|Texas Instruments Incorporated
|High-Speed Differential Line Tranceivers
|IBIS Model for SN65LVDM1676 and SN65LVDM1677
|Valid for datarates upto 650Mbps for transmitters and 200Mbps for Receivers
|Marketing part#   Voltage Range   Package-type   #pins/pkg-type
|SN65LVDM1676DGG   3.0V - 3.6V   TSSOP   64-pin(DGG) TSSOP
|SN65LVDM1676DGGG4   3.0V - 3.6V   TSSOP   64-pin(DGG) TSSOP
|SN65LVDM1676DGGR   3.0V - 3.6V   TSSOP   64-pin(DGG) TSSOP
|SN65LVDM1676DGGRG4   3.0V - 3.6V   TSSOP   64-pin(DGG) TSSOP
|SN65LVDM1677DGG   3.0V - 3.6V   TSSOP   64-pin(DGG) TSSOP
|SN65LVDM1677DGGG4   3.0V - 3.6V   TSSOP   64-pin(DGG) TSSOP
|SN65LVDM1677DGGR   3.0V - 3.6V   TSSOP   64-pin(DGG) TSSOP
|SN65LVDM1677DGGRG4   3.0V - 3.6V   TSSOP   64-pin(DGG) TSSOP
[IBIS Ver]   4.0
[File name]   sn65lvdm1676_77.ibs
[File Rev]   1.1
[Date]   01/30/2009
[Source]   Texas Instruments Incorporated.
   Analog-eLab, HPA
   12500 TI Blvd
   Dallas, TX -75243
   For Support e-mail: elab_ibis@list.ti.com
[Notes]   Revision History
   Rev 2.0: 05/09/2006
   - Initial Revision not matched to silicon
   - Revision to correct DC end points
   Rev 1.1: 01/30/2009
   - Revision is numbered down to 1.1, to comply with IBIS
   standard way of 1.x for models that are not matched to silicon
   - Models included for all the three corners
   - Models valid for SN65LVD1676 and SN65LVDM1677
   - Updated timing specficatio values for DIFF_BI and TTL_BI models
[Disclaimer] This model is designed as an aid for customers of Texas Instruments.
 TI and its licensors and suppliers make no warranties, either expressed
 or implied, with respect to this  model, including the warranties of
 merchantability or fitness for a particular purpose.
 The model is provided solely on an "as is" basis. The entire risk as to
 its quality and performance is with the customer.
[Copyright] (C)Copyright 2009 Texas Instruments Incorporated. All rights reserved.
|   SN65LVDM1676DGG, with no termination between xxY and xxZ
[Component]   SN65LVDM1676DGG
[Manufacturer]  Texas Instruments Incorporated
[Package]   |64-pin TSSOP
|   typ   min   max
R_pkg   0.3357   0.2722   0.3992
L_pkg   3.6063nH   2.3128nH   4.8998nH
C_pkg   0.7109pF   0.3688pF   1.0529pF
[Pin] signal_name  model_name   R_pin   L_pin   C_pin
 1   GND   GND   0.22128  4.47324nH  1.01397pF
 2   VCC   POWER   0.38744  4.54017nH  1.04184pF
 3   VCC   POWER   0.38686  4.26675nH  0.93417pF
 4   GND   GND   0.38300  3.98994nH  0.83251pF
 5   ATX/RX   ENABLE   0.38411  3.73937nH  0.73901pF
 6   A1A   TTL_BI   0.38160  3.47970nH  0.64411pF
 7   A2A   TTL_BI   0.37105  3.18719nH  0.49035pF
 8   A3A   TTL_BI   0.33642  2.84375nH  0.45074pF
 9   A4A   TTL_BI   0.30420  2.59359nH  0.45718pF
10   BTX/RX   ENABLE   0.30070  2.55030nH  0.46530pF
11   B1A   TTL_BI   0.27412  2.38775nH  0.44423pF
12   B2A   TTL_BI   0.28316  2.43458nH  0.43792pF
13   B3A   TTL_BI   0.28981  2.46842nH  0.44090pF
14   B4A   TTL_BI   0.28000  2.36957nH  0.41787pF
15   GND   GND   0.27427  2.26725nH  0.40273pF
16   VCC   POWER   0.27344  2.24702nH  0.36695pF
17   VCC   POWER   0.27230  2.24050nH  0.36679pF
18   GND   GND   0.27273  2.25890nH  0.40223pF
19   C1A   TTL_BI   0.27551  2.34562nH  0.41523pF
20   C2A   TTL_BI   0.27964  2.41073nH  0.43742pF
21   C3A   TTL_BI   0.27218  2.37082nH  0.43941pF
22   C4A   TTL_BI   0.28848  2.47629nH  0.45088pF
23   CTX/RX   ENABLE   0.30740  2.59389nH  0.46881pF
24   D1A   TTL_BI   0.34088  2.82097nH  0.46717pF
25   D2A   TTL_BI   0.34051  2.87482nH  0.44992pF
26   D3A   TTL_BI   0.37271  3.20165nH  0.49086pF
27   D4A   TTL_BI   0.37589  3.44878nH  0.64437pF
28   DTX/RX   ENABLE   0.37739  3.70266nH  0.74218pF
29   GND   GND   0.37850  3.96797nH  0.83809pF
30   VCC   POWER   0.38033  4.23320nH  0.94059pF
31   VCC   POWER   0.38354  4.52417nH  1.05059pF
32   GND   GND   0.21987  4.45173nH  1.01894pF
33   D4Z   DIFF_BI   0.38723  4.87938nH  0.97220pF
34   D4Y   DIFF_BI   0.38394  4.52468nH  1.04044pF
35   D3Z   DIFF_BI   0.38248  4.24575nH  0.93538pF
36   D3Y   DIFF_BI   0.38370  3.99984nH  0.83632pF
37   D2Z   DIFF_BI   0.38672  3.76077nH  0.74367pF
38   D2Y   DIFF_BI   0.39239  3.55100nH  0.65111pF
39   D1Z   DIFF_BI   0.38504  3.27768nH  0.49727pF
40   D1Y   DIFF_BI   0.31818  2.73755nH  0.44436pF
41   C4Z   DIFF_BI   0.32127  2.70100nH  0.45913pF
42   C4Y   DIFF_BI   0.31115  2.61731nH  0.46671pF
43   C3Z   DIFF_BI   0.30136  2.55465nH  0.45112pF
44   C3Y   DIFF_BI   0.29406  2.50298nH  0.44285pF
45   C2Z   DIFF_BI   0.29101  2.47812nH  0.44091pF
46   C2Y   DIFF_BI   0.28926  2.42717nH  0.41837pF
47   C1Z   DIFF_BI   0.28865  2.35505nH  0.40495pF
48   C1Y   DIFF_BI   0.28916  2.34232nH  0.36962pF
49   B4Z   DIFF_BI   0.28633  2.32500nH  0.36878pF
50   B4Y   DIFF_BI   0.28177  2.31280nH  0.40298pF
51   B3Z   DIFF_BI   0.27796  2.35941nH  0.41458pF
52   B3Y   DIFF_BI   0.27453  2.37863nH  0.43615pF
53   B2Z   DIFF_BI   0.27226  2.36951nH  0.43902pF
54   B2Y   DIFF_BI   0.27640  2.40099nH  0.44636pF
55   B1Z   DIFF_BI   0.29100  2.49139nH  0.46130pF
56   B1Y   DIFF_BI   0.29972  2.56747nH  0.45350pF
57   A4Z   DIFF_BI   0.32271  2.76232nH  0.44507pF
58   A4Y   DIFF_BI   0.39212  3.31525nH  0.49929pF
59   A3Z   DIFF_BI   0.39916  3.58578nH  0.65712pF
60   A3Y   DIFF_BI   0.39255  3.78985nH  0.75190pF
61   A2Z   DIFF_BI   0.38864  4.02433nH  0.84518pF
62   A2Y   DIFF_BI   0.38679  4.26678nH  0.94612pF
63   A1Z   DIFF_BI   0.38755  4.54277nH  1.05293pF
64   A1Y   DIFF_BI   0.39081  4.89981nH  0.97900pF
[Diff_pin]   inv_pin   vdiff   tdelay_typ   tdelay_min   tdelay_max
| The 'xxY' pin is diff_pin and the 'xxZ' pin is the inv_pin
34   33   100mV   0   0   0
36   35   100mV   0   0   0
38   37   100mV   0   0   0
40   39   100mV   0   0   0
42   41   100mV   0   0   0
44   43   100mV   0   0   0
46   45   100mV   0   0   0
48   47   100mV   0   0   0
50   49   100mV   0   0   0
52   51   100mV   0   0   0
54   53   100mV   0   0   0
56   55   100mV   0   0   0
58   57   100mV   0   0   0
60   59   100mV   0   0   0
62   61   100mV   0   0   0
64   63   100mV   0   0   0
|   SN65LVDM1677DGG, with 100 Ohm termination between xxY and xxZ
[Component]   SN65LVDM1677DGG
[Manufacturer]  Texas Instruments Incorporated
[Package]   |64-pin TSSOP
|   typ   min   max
R_pkg   0.3357   0.2722   0.3992
L_pkg   3.6063nH   2.3128nH   4.8998nH
C_pkg   0.7109pF   0.3688pF   1.0529pF
[Pin] signal_name  model_name   R_pin   L_pin   C_pin
 1   GND   GND   0.22128  4.47324nH  1.01397pF
 2   VCC   POWER   0.38744  4.54017nH  1.04184pF
 3   VCC   POWER   0.38686  4.26675nH  0.93417pF
 4   GND   GND   0.38300  3.98994nH  0.83251pF
 5   ATX/RX   ENABLE   0.38411  3.73937nH  0.73901pF
 6   A1A   TTL_BI   0.38160  3.47970nH  0.64411pF
 7   A2A   TTL_BI   0.37105  3.18719nH  0.49035pF
 8   A3A   TTL_BI   0.33642  2.84375nH  0.45074pF
 9   A4A   TTL_BI   0.30420  2.59359nH  0.45718pF
10   BTX/RX   ENABLE   0.30070  2.55030nH  0.46530pF
11   B1A   TTL_BI   0.27412  2.38775nH  0.44423pF
12   B2A   TTL_BI   0.28316  2.43458nH  0.43792pF
13   B3A   TTL_BI   0.28981  2.46842nH  0.44090pF
14   B4A   TTL_BI   0.28000  2.36957nH  0.41787pF
15   GND   GND   0.27427  2.26725nH  0.40273pF
16   VCC   POWER   0.27344  2.24702nH  0.36695pF
17   VCC   POWER   0.27230  2.24050nH  0.36679pF
18   GND   GND   0.27273  2.25890nH  0.40223pF
19   C1A   TTL_BI   0.27551  2.34562nH  0.41523pF
20   C2A   TTL_BI   0.27964  2.41073nH  0.43742pF
21   C3A   TTL_BI   0.27218  2.37082nH  0.43941pF
22   C4A   TTL_BI   0.28848  2.47629nH  0.45088pF
23   CTX/RX   ENABLE   0.30740  2.59389nH  0.46881pF
24   D1A   TTL_BI   0.34088  2.82097nH  0.46717pF
25   D2A   TTL_BI   0.34051  2.87482nH  0.44992pF
26   D3A   TTL_BI   0.37271  3.20165nH  0.49086pF
27   D4A   TTL_BI   0.37589  3.44878nH  0.64437pF
28   DTX/RX   ENABLE   0.37739  3.70266nH  0.74218pF
29   GND   GND   0.37850  3.96797nH  0.83809pF
30   VCC   POWER   0.38033  4.23320nH  0.94059pF
31   VCC   POWER   0.38354  4.52417nH  1.05059pF
32   GND   GND   0.21987  4.45173nH  1.01894pF
33   D4Z   DIFF_BI   0.38723  4.87938nH  0.97220pF
34   D4Y   DIFF_BI   0.38394  4.52468nH  1.04044pF
35   D3Z   DIFF_BI   0.38248  4.24575nH  0.93538pF
36   D3Y   DIFF_BI   0.38370  3.99984nH  0.83632pF
37   D2Z   DIFF_BI   0.38672  3.76077nH  0.74367pF
38   D2Y   DIFF_BI   0.39239  3.55100nH  0.65111pF
39   D1Z   DIFF_BI   0.38504  3.27768nH  0.49727pF
40   D1Y   DIFF_BI   0.31818  2.73755nH  0.44436pF
41   C4Z   DIFF_BI   0.32127  2.70100nH  0.45913pF
42   C4Y   DIFF_BI   0.31115  2.61731nH  0.46671pF
43   C3Z   DIFF_BI   0.30136  2.55465nH  0.45112pF
44   C3Y   DIFF_BI   0.29406  2.50298nH  0.44285pF
45   C2Z   DIFF_BI   0.29101  2.47812nH  0.44091pF
46   C2Y   DIFF_BI   0.28926  2.42717nH  0.41837pF
47   C1Z   DIFF_BI   0.28865  2.35505nH  0.40495pF
48   C1Y   DIFF_BI   0.28916  2.34232nH  0.36962pF
49   B4Z   DIFF_BI   0.28633  2.32500nH  0.36878pF
50   B4Y   DIFF_BI   0.28177  2.31280nH  0.40298pF
51   B3Z   DIFF_BI   0.27796  2.35941nH  0.41458pF
52   B3Y   DIFF_BI   0.27453  2.37863nH  0.43615pF
53   B2Z   DIFF_BI   0.27226  2.36951nH  0.43902pF
54   B2Y   DIFF_BI   0.27640  2.40099nH  0.44636pF
55   B1Z   DIFF_BI   0.29100  2.49139nH  0.46130pF
56   B1Y   DIFF_BI   0.29972  2.56747nH  0.45350pF
57   A4Z   DIFF_BI   0.32271  2.76232nH  0.44507pF
58   A4Y   DIFF_BI   0.39212  3.31525nH  0.49929pF
59   A3Z   DIFF_BI   0.39916  3.58578nH  0.65712pF
60   A3Y   DIFF_BI   0.39255  3.78985nH  0.75190pF
61   A2Z   DIFF_BI   0.38864  4.02433nH  0.84518pF
62   A2Y   DIFF_BI   0.38679  4.26678nH  0.94612pF
63   A1Z   DIFF_BI   0.38755  4.54277nH  1.05293pF
64   A1Y   DIFF_BI   0.39081  4.89981nH  0.97900pF
[Diff_pin]   inv_pin   vdiff   tdelay_typ   tdelay_min   tdelay_max
| The 'xxY' pin is diff_pin and the 'xxZ' pin is the inv_pin
34   33   100mV   0   0   0
36   35   100mV   0   0   0
38   37   100mV   0   0   0
40   39   100mV   0   0   0
42   41   100mV   0   0   0
44   43   100mV   0   0   0
46   45   100mV   0   0   0
48   47   100mV   0   0   0
50   49   100mV   0   0   0
52   51   100mV   0   0   0
54   53   100mV   0   0   0
56   55   100mV   0   0   0
58   57   100mV   0   0   0
60   59   100mV   0   0   0
62   61   100mV   0   0   0
64   63   100mV   0   0   0
[series pin mapping]  pin_2   model_name
34   33   series100
36   35   series100
38   37   series100
40   39   series100
42   41   series100
44   43   series100
46   45   series100
48   47   series100
50   49   series100
52   51   series100
54   53   series100
56   55   series100
58   57   series100
60   59   series100
62   61   series100
64   63   series100
[Model]   series100
Model_type   Series
|   typ   min   max
C_comp   0pF   0pF   0pF
[Voltage Range]   3.3V   3.0V   3.6V
[Pullup Reference]   3.3V   3.0V   3.6V
| Junction Temperature (Ambient temp is 25C typ, 85C min, -40C max)
[Temperature Range]   40.0   100.0   -40.0
[R series]   100   88   132
| Models and submodels in the file (4): series100 (Series), ENABLE (Input), DIFF_BI (I/O), TTL_BI (3-state)
